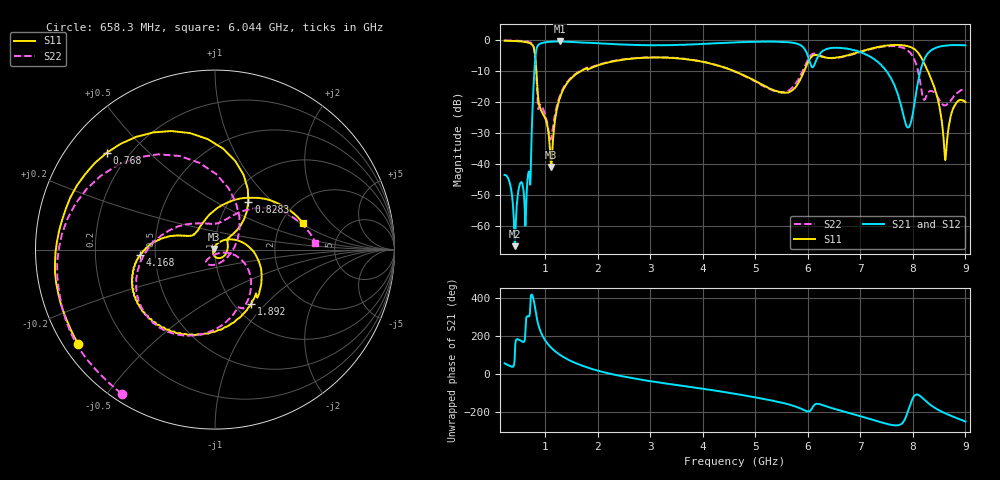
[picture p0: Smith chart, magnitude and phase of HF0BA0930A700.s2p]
!Agilent Technologies,E8358A,US41080443,A.07.50.56
!Agilent E8358A: A.07.50.56
!Date: Monday, March 28, 2016 12:57:16
!Correction: S11(Full 2 Port(1,2))
!S21(Full 2 Port(1,2))
!S12(Full 2 Port(1,2))
!S22(Full 2 Port(1,2))
!S2P File: Measurements: S11, S21, S12, S22:
# Hz S  dB  R 50
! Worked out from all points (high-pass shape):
!   1601 points, 225 MHz to 9 GHz, reference 50 ohm
!   highest |S21| = -0.36 dB at 1.273 GHz (marker M1); lowest = -66.5 dB at 422.4 MHz (marker M2)
!   |S21| within 3 dB of the highest: 826.1 MHz to 5.957 GHz (5.131 GHz wide, 151 % of centre); 8.336 GHz to end of sweep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
!   lowest |S11| = -40.9 dB at 1.113 GHz (marker M3), VSWR 1.02, Z = 49.2 + j0.342 ohm
!   |S11| at or under -10 dB: 829.3 MHz to 1.672 GHz (842.7 MHz wide, 67.4 % of centre); 4.601 GHz to 5.927 GHz (1.327 GHz wide, 25.2 % of centre); 8.286 GHz to end of sweep
!   |S22| runs from -32.1 to 0.0 dB; largest |S21 - S12| = 0.014
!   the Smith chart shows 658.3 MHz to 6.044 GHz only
!   S11 on the Smith chart (normalised r, x): 658.3 MHz: 0.04, -0.31; 768 MHz: 0.12, +0.38; 828.3 MHz: 1.22, +0.73; 1.892 GHz: 1.19, -0.83; 4.168 GHz: 0.41, -0.03; 6.044 GHz: 2.63, +1.04
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2.25e8  -0.11 -36.2  -43.49 55.6  -43.59 55.9  -0.03 -31.7
4.224375e8  -0.23 -73.6  -66.53 123.9  -66.74 121.6  -0.11 -63.6
6.582656e8  -0.66 -145.5  -45.58 -57.2  -45.71 -57.3  -0.39 -123.0
7.679531e8  -1.84 138.2  -17.83 39.4  -17.92 39.6  -1.51 168.3
8.282812e8  -9.73 55.2  -3.15 -51.7  -3.25 -51.6  -10.86 66.0
9.544219e8  -23.75 -19.1  -0.77 -163.4  -0.87 -163.2  -21.99 -127.7
1.113469e9  -40.88 157.4  -0.42 137.6  -0.53 137.7  -31.56 -55.2
1.272516e9  -18.87 29.7  -0.36 101.4  -0.48 101.6  -18.12 -16.6
1.689328e9  -9.82 -37.2  -0.69 45.0  -0.79 45.1  -9.63 -55.5
1.89225e9  -8.76 -56.5  -0.81 25.8  -0.91 25.9  -8.55 -73.7
3.153656e9  -5.54 -138.0  -1.59 -44.5  -1.70 -44.4  -5.47 -130.6
4.168266e9  -7.58 -175.8  -1.00 -84.7  -1.09 -84.6  -7.55 -171.1
4.6125e9  -10.06 169.8  -0.67 -104.0  -0.76 -103.9  -10.08 166.1
5.692922e9  -16.25 122.0  -0.73 -164.6  -0.84 -164.4  -15.49 73.1
6.043922e9  -5.81 16.5  -7.27 166.8  -7.40 166.8  -5.03 4.0
6.076828e9  -5.19 1.8  -8.64 178.6  -8.73 178.8  -4.54 -8.3
6.778828e9  -4.78 -111.1  -2.83 155.5  -2.93 155.6  -4.89 -122.3
7.541156e9  -1.66 -175.1  -11.10 95.3  -11.19 95.6  -1.91 157.9
7.914094e9  -1.93 141.6  -28.14 170.7  -28.31 171.1  -3.46 93.6
8.215734e9  -7.43 91.6  -6.13 -134.8  -6.26 -134.6  -19.23 -98.0
8.616094e9  -38.71 142.5  -1.70 153.3  -1.80 153.4  -21.02 -174.1
9e9  -19.98 -163.4  -1.62 110.3  -1.72 110.4  -15.73 -133.7
